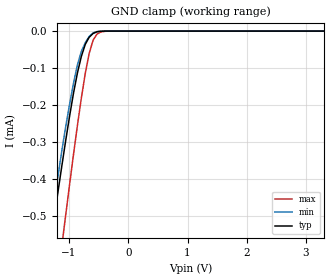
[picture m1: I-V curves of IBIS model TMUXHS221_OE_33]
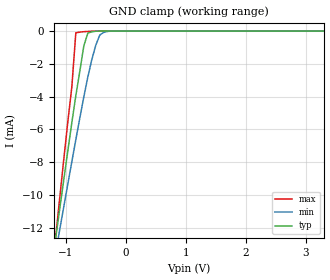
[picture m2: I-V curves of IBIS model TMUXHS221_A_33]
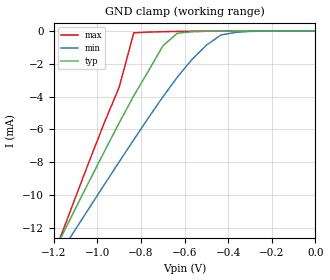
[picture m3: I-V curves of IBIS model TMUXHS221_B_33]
| TEXAS INSTRUMENTS INCORPORATED
| Standard Linear and Logic Group
| IBIS Model of TMUXHS221
|  USB2.0 480Mbps switch
|  2:1 Multiplexer/Demultiplexer
| This file contains package information for the following:
|  UQFN 10-pin (NKG) package as [Component] TMUXHS221
| This device can be powered at the following Vccs:
|  3.3 volt Vcc
| This file provides unique models under the [Model Selector] for each Vcc.
| For operation at a specific Vcc, select the appropriate model after each
| [Model Selector] keyword.
[IBIS Ver]   3.2
[Comment char]  |_char
[File Name]   tmuxhs221.ibs
[File Rev]   1.2 | a_die
[Date]   March 22, 2005
[Source]   Data created from TI-SPICE simulations at TI-SLL.
[Notes]   The following is an IBIS list for the TS5A3154.
   Please contact sllibis@ti.com with questions and
   comments concerning SLL IBIS models.
   - FILE REV HISTORY
   - 1.1 Release IBIS file on 03/23/05
   - 1.2 Package data updated 12/20/07
   - Power clamp data deleted in OE, switch as there is
   is no power-clamp diode.
   - Non-monotonic data due to FET characteristics.
   - NCH MOSFET, so [Series Mosfet] model can have rising
   or falling currents
[Disclaimer] Property of Texas Instruments Incorporated.  Unauthorized
   reproduction and/or distribution is strictly prohibited.
   This product is protected under copyright law.
   Created  2005, (C) Copyright  2005, Texas Instruments
   Incorporated, All Rights Reserved
   UNLESS THERE IS A SIGNED, WRITTEN AGREEMENT TO THE
   CONTRARY, TEXAS INSTRUMENTS (TI) IS PROVIDING THE IBIS
   MODELS  AND WITHOUT ANY WARRANTY, EXPRESSED OR
   IMPLIED.  TI assumes no liability for:
   1) the accuracy of the IBIS models provided to your
   company;
   2) the proper functioning of these IBIS Models in your
   design or for any resulting applications; or
   3) infringement of patents, copyrights or intellectual
   property rights resulting from your use of these IBIS
   models.
   TI provides IBIS Models as a service to our customers.
   You and your company shall not distribute, sell or give
   these models to anyone else without prior written
   permission from TI.
   TI reserves the right to make changes to our products or
   to discontinue any semiconductor product or service
   without notice, and advises our customers to obtain the
   latest version of relevant information to verify, before
   placing orders, that the information being relied on is
   current.
   Please be aware that your receipt and use of the IBIS
   information provided shall serve as acceptance of these
   terms and conditions.  If you do not accept these terms,
   you should return or destroy the IBIS models and any
   other accompanying information immediately.
| Component TMUXHS221 10-pin NKG
[Component]   TMUXHS221
[Manufacturer]   Texas Instruments, Inc.
[Package]
|   typ   min   max
R_pkg   1.000e-03   1.000e-03   4.000e-03
L_pkg   6.400e-11   2.400e-11   3.790e-10
C_pkg   5.800e-14   0.000e+00   6.700e-14
[Pin]   signal_name   model_name   R_pin   L_pin   C_pin
1   D+   TMUXHS221_A   1.000e-03   2.500e-11   6.400e-14
2   D-   TMUXHS221_A   1.000e-03   2.400e-11   6.700e-14
3   GND   GND   1.000e-03   2.400e-11   6.700e-14
4   DA-   TMUXHS221_B   1.000e-03   2.500e-11   6.400e-14
5   DA+   TMUXHS221_B   1.000e-03   2.500e-11   6.400e-14
6   DB-   TMUXHS221_B   1.000e-03   2.400e-11   6.700e-14
7   DB+   TMUXHS221_B   1.000e-03   2.400e-11   6.700e-14
8   OEn   TMUXHS221_OE   1.000e-03   2.500e-11   6.400e-14
9   DB+   TMUXHS221_B   1.000e-03   2.400e-11   6.700e-14
10   SEL   TMUXHS221_OE   1.000e-03   2.500e-11   6.400e-14
[Series Switch Groups]
| Function Group States
On  1 /   | D+->DA+ D-->DA- OEn LOW SEL LOW
On  2 /   | D+->DB+ D-->DB- OEn LOW SEL HIGH
On  3 /   | DA+->D+ DA-->D- OEn LOW SEL LOW
On  4 /   | DB+->D+ DB-->D- OEn LOW SEL HIGH
Off 1 3 /   | OEn LOW SEL HIGH
Off 2 4 /   | OEn LOW SEL LOW
Off 1 2 3 4 /   | OEn HIGH
[Series Pin Mapping]   pin_2   model_name   function_table_group
1   5   TMUXHS221_A_S   1
1   7   TMUXHS221_A_S   2
5   1   TMUXHS221_B_S   3
7   1   TMUXHS221_B_S   4
| Model TMUXHS221_OE
[Model Selector]   TMUXHS221_OE
TMUXHS221_OE_33   3.3 volt Vcc
| Model TMUXHS221_A
[Model Selector]   TMUXHS221_A
TMUXHS221_A_33   3.3 volt Vcc
| Model TMUXHS221_A_S
[Model Selector]   TMUXHS221_A_S
TMUXHS221_A_33_S   3.3 volt Vcc_S
| Model TMUXHS221_B
[Model Selector]   TMUXHS221_B
TMUXHS221_B_33   3.3 volt Vcc
| Model TMUXHS221_B_S
[Model Selector]   TMUXHS221_B_S
TMUXHS221_B_33_S   3.3 volt Vcc_S
[Model]   TMUXHS221_A_33_S
Model_type  Series_switch
| variable   typ   min   max
C_comp   0   0   0
[Temperature Range]   27   125   -40
| Ambient temperature   27   125   -40
[Voltage range]   3.3   3   3.6
[On]
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[Off]
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[Model]   TMUXHS221_B_33_S
Model_type  Series_switch
| variable   typ   min   max
C_comp   0   0   0
[Temperature Range]   27   125   -40
| Ambient temperature   27   125   -40
[Voltage range]   3.3   3   3.6
[On]
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[Off]
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| Models and submodels in the file (5): TMUXHS221_OE_33 (Input), TMUXHS221_A_33_S (Series_switch), TMUXHS221_A_33 (Terminator), TMUXHS221_B_33_S (Series_switch), TMUXHS221_B_33 (Terminator)
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[Model]   TMUXHS221_OE_33
Model_type  Input
Vinl=0.4
Vinh=1.4
| variable   typ   min   max
C_comp   4.72pF   4.37pF   5.12pF
[Temperature Range]   27   125   -40
| Ambient temperature   27   125   -40
[Voltage range]   3.3   3   3.6
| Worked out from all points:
|   GND clamp passes 1 mA (typ) near -1.69 V on its own axis
[GND Clamp]
| TS5A3154_OE_33
|Voltage   I(typ)   I(min)   I(max)
-3.3V     -2.885mA   -3.04mA    -3.546mA
-1.32V    -580.7uA   -542.5uA   -838.5uA
-1.254V   -507.4uA   -466.1uA   -751.6uA
-1.122V   -364uA     -322.7uA   -579.9uA
-1.056V   -294.8uA   -257.6uA   -495.6uA
-858mV    -112.5uA   -90.5uA    -253.8uA
-726mV    -35.8uA    -31.3uA    -114.1uA
-660mV    -16.6uA    -14.7uA    -60.1uA
-594mV    -6.42uA    -4.97uA    -24.6uA
-528mV    -1.94uA    -1.21uA    -7.98uA
-330mV    -17.3nA    -2.97nA    -160nA
3.3V      20.1pA     16.5pA     2.38nA
[Model]   TMUXHS221_A_33
Model_type  Terminator
| variable   typ   min   max
C_comp   2.7pF   3.5pF   2.4pF
| C_tri-state   2.7pF   3.5pF   2.4pF
[Temperature Range]   27   125   -40
| Ambient temperature   27   125   -40
[Voltage range]   3.3   3   3.6
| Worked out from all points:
|   GND clamp passes 1 mA (typ) near -0.70 V on its own axis
[GND Clamp]
| TMUXHS221_A_33
|   Voltage   I(typ)   I(min)   I(max)
-3.3V     -71.21mA   -59.24mA   -90.56mA
-1.167V   -12.58mA   -13.47mA   -12.47mA
-1.1V     -10.81mA   -12.08mA   -10.12mA
-966.7mV  -7.31mA    -9.334mA   -5.535mA
-900mV    -5.596mA   -7.974mA   -3.415mA
-833.3mV  -3.943mA   -6.628mA   -107.4uA
-700mV    -906.2uA   -4.017mA   -37.4uA
-633.3mV  -127.8uA   -2.805mA   -20.5uA
-500mV    -9.78uA    -857.7uA   -2.65uA
-433.3mV  -1.75uA    -237.3uA   -581nA
-366.7mV  -311nA     -79.2uA    -95.4nA
3.3V      89.2pA     726pA      85.4pA
[Model]   TMUXHS221_B_33
Model_type  Terminator
| variable   typ   min   max
C_comp   1.7pF   2.5pF   1.4pF
| C_tri-state   1.7pF   2.5pF   1.4pF
[Temperature Range]   27   125   -40
| Ambient temperature   27   125   -40
[Voltage range]   3.3   3   3.6
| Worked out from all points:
|   GND clamp passes 1 mA (typ) near -0.70 V on its own axis
[GND Clamp]
| TMUXHS221_B_33
|   Voltage   I(typ)   I(min)   I(max)
-3.3V     -71.21mA   -59.24mA   -90.56mA
-1.167V   -12.58mA   -13.47mA   -12.47mA
-1.1V     -10.81mA   -12.08mA   -10.12mA
-966.7mV  -7.31mA    -9.334mA   -5.535mA
-900mV    -5.596mA   -7.974mA   -3.415mA
-833.3mV  -3.943mA   -6.628mA   -107.4uA
-700mV    -906.2uA   -4.017mA   -37.4uA
-633.3mV  -127.8uA   -2.805mA   -20.5uA
-500mV    -9.78uA    -857.7uA   -2.65uA
-433.3mV  -1.75uA    -237.3uA   -581nA
-300mV    -53.2nA    -17.7uA    -11nA
0V        -22.3pA    -4.41nA    -7.33pA
